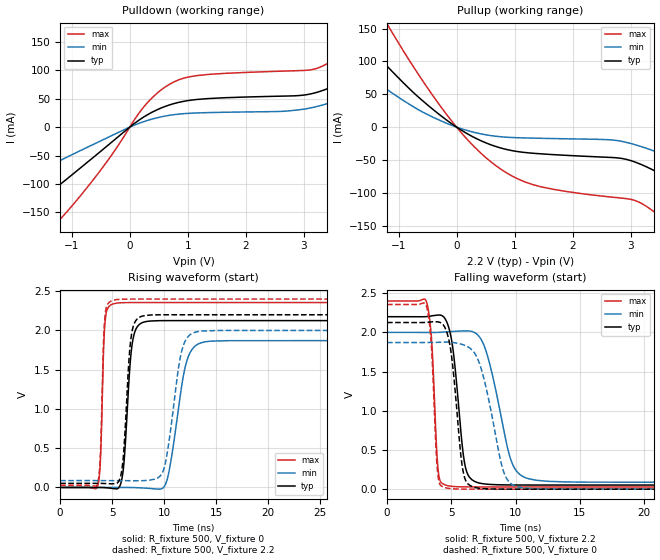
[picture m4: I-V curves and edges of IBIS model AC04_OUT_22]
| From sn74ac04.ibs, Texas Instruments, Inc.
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[Model]   AC04_OUT_22
Model_type  Output
Vref =   0
Rref =   500
Cref =   50p
Vmeas =   1.1
| variable   typ   min   max
C_comp   11.09pF   7.15pF   16.36pF
| C_pullup   10.49pF   7.22pF   12.81pF
| C_pulldown   11.68pF   7.15pF   16.36pF
[Temperature Range]   40   100   -40
| Ambient temperature   25   85   -40
[Voltage range]   2.2   2   2.4
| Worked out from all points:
|   slope of the pulldown table from 0 to 0.33 V, typ, clamps not added: 14.2 ohm
|   slope of the pullup table from 0 to 0.33 V, typ, clamps not added: 19.5 ohm
|   rising waveform, R_fixture 500, V_fixture 0: 20-80 % time 612ps typ, 1.27ns min, 307ps max; typ from 0 V to 2.13 V
|   falling waveform, R_fixture 500, V_fixture 2.2: 20-80 % time 761ps typ, 1.5ns min, 405ps max; typ from 2.2 V to 0.052 V
|   rising waveform, R_fixture 500, V_fixture 2.2: 20-80 % time 577ps typ, 1.16ns min, 301ps max; typ from 0.052 V to 2.2 V
|   falling waveform, R_fixture 500, V_fixture 0: 20-80 % time 731ps typ, 1.43ns min, 399ps max; typ from 2.13 V to 0 V
[Pulldown]
| AC04_OUT_22
|   Voltage   I(typ)   I(min)   I(max)
-5V       -399.5mA   -251.5mA   -506.5mA
-3.795V   -304.4mA   -189.2mA   -397.8mA
-2.38V    -195.3mA   -117.7mA   -273.3mA
-1.37V    -114.8mA   -67.2mA    -180.3mA
260mV     19.01mA    10.32mA    37.75mA
630mV     37.18mA    19.86mA    71.96mA
1.155V    48.67mA    24.97mA    90.68mA
3.23V     61.34mA    36.36mA    103.6mA
4.245V    112.9mA    74.79mA    179.3mA
5.045V    172.8mA    117.7mA    268.3mA
6.075V    265.3mA    183mA      403.8mA
10V       715.8mA    477.6mA    1.076A
[Pullup]
| AC04_OUT_22
|   Voltage   I(typ)   I(min)   I(max)
-5V       513.6mA    327.7mA    841.6mA
-2.71V    244.6mA    157mA      399.7mA
-1.835V   153.8mA    97.19mA    254.6mA
-1.285V   100.8mA    62.27mA    169.8mA
-150mV    9.277mA    5.032mA    16.72mA
760mV     -31.71mA   -14.62mA   -63.83mA
1.415V    -40.4mA    -16.93mA   -89.92mA
2.87V     -48.02mA   -22.07mA   -108.3mA
3.815V    -86.49mA   -50.4mA    -158.2mA
4.9V      -153.4mA   -94.99mA   -246.4mA
6.355V    -256.5mA   -163.1mA   -371.4mA
10V       -543.6mA   -351.9mA   -704mA
[Ramp]
| AC04_OUT_22
| variable   typ   min   max
dV/dt_r   1.29/6.23E-10   1.14/1.28E-09   1.42/3.21E-10
dV/dt_f   1.30/7.76E-10   1.16/1.52E-09   1.44/4.14E-10
R_load = 500
[Rising Waveform]
| AC04_OUT_22
R_fixture =   500
C_fixture =   0
L_fixture =   0
V_fixture =   0
V_fixture_min = 0
V_fixture_max = 0
|   Time   V(typ)   V(min)   V(max)
0s        1.052nV    1.968nV    536.1pV
3.63ns    129.8uV    138.5uV    24.43mV
4.31ns    -2.607mV   130.8uV    2.09V
5.065ns   -13.41mV   132.3uV    2.337V
5.955ns   117.8mV    93.17uV    2.353V
6.91ns    1.807V     -1.092mV   2.355V
7.985ns   2.104V     -6.891mV   2.356V
10.18ns   2.125V     52.63mV    2.356V
13.54ns   2.126V     1.842V     2.356V
50ns      2.126V     1.871V     2.356V
[Falling Waveform]
| AC04_OUT_22
R_fixture =   500
C_fixture =   0
L_fixture =   0
V_fixture =   2.2
V_fixture_min = 2
V_fixture_max = 2.4
|   Time   V(typ)   V(min)   V(max)
0s        2.2V       2V         2.4V
3.08ns    2.201V     1.999V     2.385V
3.46ns    2.21V      1.999V     1.92V
3.985ns   2.221V     2V         232.5mV
4.655ns   2.13V      2.007V     47.26mV
6.06ns    310.2mV    2.019V     29.14mV
7.095ns   81.67mV    1.961V     28.31mV
9.655ns   53.72mV    364.1mV    28.17mV
11.06ns   52.76mV    131mV      28.17mV
50ns      52.46mV    87.4mV     28.17mV
[Rising Waveform]
| AC04_OUT_22
R_fixture =   500
C_fixture =   0
L_fixture =   0
V_fixture =   2.2
V_fixture_min = 2
V_fixture_max = 2.4
|   Time   V(typ)   V(min)   V(max)
0s        52.46mV    87.4mV     28.17mV
3.615ns   52.3mV     87.47mV    55.87mV
4.295ns   50.14mV    87.29mV    2.154V
5.01ns    46.5mV     87.1mV     2.381V
5.91ns    199.9mV    86.85mV    2.398V
6.805ns   1.89V      86.13mV    2.4V
7.805ns   2.179V     85.89mV    2.4V
9.945ns   2.2V       219.8mV    2.4V
12.92ns   2.2V       1.975V     2.4V
50ns      2.2V       2V         2.4V
[Falling Waveform]
| AC04_OUT_22
R_fixture =   500
C_fixture =   0
L_fixture =   0
V_fixture =   0
V_fixture_min = 0
V_fixture_max = 0
|   Time   V(typ)   V(min)   V(max)
0s        2.126V     1.871V     2.356V
3.065ns   2.127V     1.871V     2.336V
3.445ns   2.134V     1.871V     1.844V
3.935ns   2.134V     1.873V     216.1mV
4.56ns    2.042V     1.876V     18.31mV
5.905ns   239.2mV    1.843V     962.7uV
6.8ns     23.31mV    1.739V     182.8uV
9.045ns   768.6uV    236.1mV    3.983uV
10.22ns   188.5uV    27.56mV    732.1nV
50ns      -3.709nV   -3.886nV   -3.065nV
